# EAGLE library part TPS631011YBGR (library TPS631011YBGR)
Switching Voltage Regulators 1.5-A output current buck-boost converter 8-DSBGA -40 to 125 Source: Datasheet
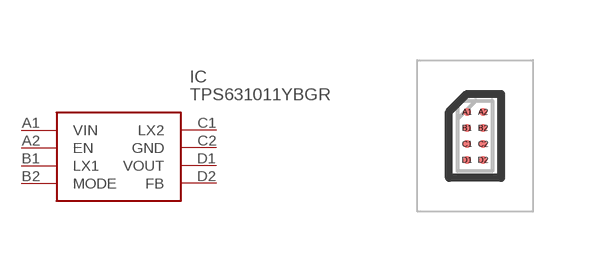
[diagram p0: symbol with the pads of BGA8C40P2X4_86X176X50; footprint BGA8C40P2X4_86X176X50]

Designator prefix IC

## TPS631011YBGR (Description: Switching Voltage Regulators 1.5-A output current buck-boost converter 8-DSBGA -40 to 125; Height: 0.5mm; Manufacturer_Name: Texas Instruments; Manufacturer_Part_Number: TPS631011YBGR; Mouser_Part_Number: 595-TPS631011YBGR; Mouser_Price-Stock: https://www.mouser.co.uk/ProductDetail/Texas-Instruments/TPS631011YBGR?qs=HoCaDK9Nz5dCMMb4Eya3qA%3D%3D)  [BGA8C40P2X4_86X176X50]
A1  VIN
A2  EN
B1  LX1
B2  MODE
C1  LX2
C2  GND
D1  VOUT
D2  FB

## Footprint BGA8C40P2X4_86X176X50 (pad centres in mm)
8-BGAeee
smd 0.2 x 0.2: A1 -0.2,0.6; A2 0.2,0.6; B1 -0.2,0.2; B2 0.2,0.2; C1 -0.2,-0.2; C2 0.2,-0.2; D1 -0.2,-0.6; D2 0.2,-0.6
